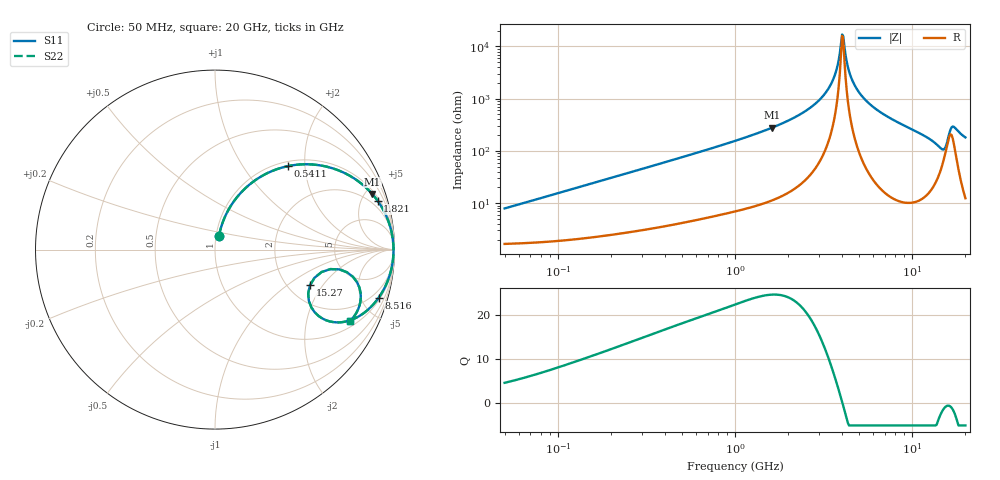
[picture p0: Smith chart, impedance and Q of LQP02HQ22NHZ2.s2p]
!Murata Part Number: LQP02HQ22NHZ2
!These Parameters are Measured in Series Mode Connection
!  o--[Z]--o
!Port1  Port2
!  o-------o
!Freq. Start=50[MHz] Stop=20[GHz], 401[Steps]
# Hz S RI R 50
!Freq.(Hz) S11(Real) S11(Imag) S21(Real) S21(Imag) S12(Real) S12(Imag) S22(Real) S22(Imag)
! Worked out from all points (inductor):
!   401 points, 50 MHz to 20 GHz, reference 50 ohm
!   read as one part in series: L = 24.6 nH near 51.52 MHz
!   highest Q = 24.7 at 1.615 GHz (marker M1), where L = 27.4 nH
!   self-resonance near 4.027 GHz
!   S11 on the Smith chart (normalised r, x): 50 MHz: 1.03, +0.15; 541.1 MHz: 1.09, +1.63; 1.821 GHz: 1.27, +6.58; 8.516 GHz: 1.22, -6.76; 15.27 GHz: 2.60, -1.52; 20 GHz: 1.25, -3.62
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5e7  0.022 0.0745  0.978 -0.0745  0.978 -0.0745  0.022 0.0745
1.364002e8  0.06 0.1925  0.94 -0.1925  0.94 -0.1925  0.06 0.1925
3.721004e8  0.2532 0.4052  0.7468 -0.4052  0.7468 -0.4052  0.2532 0.4052
5.411141e8  0.4057 0.4649  0.5943 -0.4649  0.5943 -0.4649  0.4057 0.4649
1e9  0.6996 0.4367  0.3004 -0.4367  0.3004 -0.4367  0.6996 0.4367
1.614971e9  0.8757 0.3103  0.1243 -0.3103  0.1243 -0.3103  0.8757 0.3103
1.820564e9  0.9065 0.2715  0.0935 -0.2715  0.0935 -0.2715  0.9065 0.2715
2.728004e9  0.9739 0.1347  0.0261 -0.1347  0.0261 -0.1347  0.9739 0.1347
3.519108e9  0.9917 0.048  0.00828 -0.048  0.00828 -0.048  0.9917 0.048
3.736399e9  0.9935 0.0275  0.0065 -0.0275  0.0065 -0.0275  0.9935 0.0275
4.026975e9  0.9945 0.00191  0.00553 -0.00191  0.00553 -0.00191  0.9945 0.00191
4.149438e9  0.9945 -0.00836  0.00553 0.00836  0.00553 0.00836  0.9945 -0.00836
4.472136e9  0.9935 -0.0341  0.00652 0.0341  0.00652 0.0341  0.9935 -0.0341
4.89267e9  0.9904 -0.0653  0.00961 0.0653  0.00961 0.0653  0.9904 -0.0653
5.769027e9  0.9789 -0.1234  0.0211 0.1234  0.0211 0.1234  0.9789 -0.1234
7.442007e9  0.9432 -0.2163  0.0568 0.2163  0.0568 0.2163  0.9432 -0.2163
8.516016e9  0.9125 -0.2671  0.0875 0.2671  0.0875 0.2671  0.9125 -0.2671
1.314879e10  0.6754 -0.4054  0.3246 0.4054  0.3246 0.4054  0.6754 -0.4054
1.527346e10  0.5289 -0.1993  0.4711 0.1993  0.4711 0.1993  0.5289 -0.1993
1.597544e10  0.6431 -0.1086  0.3569 0.1086  0.3569 0.1086  0.6431 -0.1086
1.696185e10  0.7908 -0.1809  0.2092 0.1809  0.2092 0.1809  0.7908 -0.1809
2e10  0.7524 -0.3987  0.2476 0.3987  0.2476 0.3987  0.7524 -0.3987
